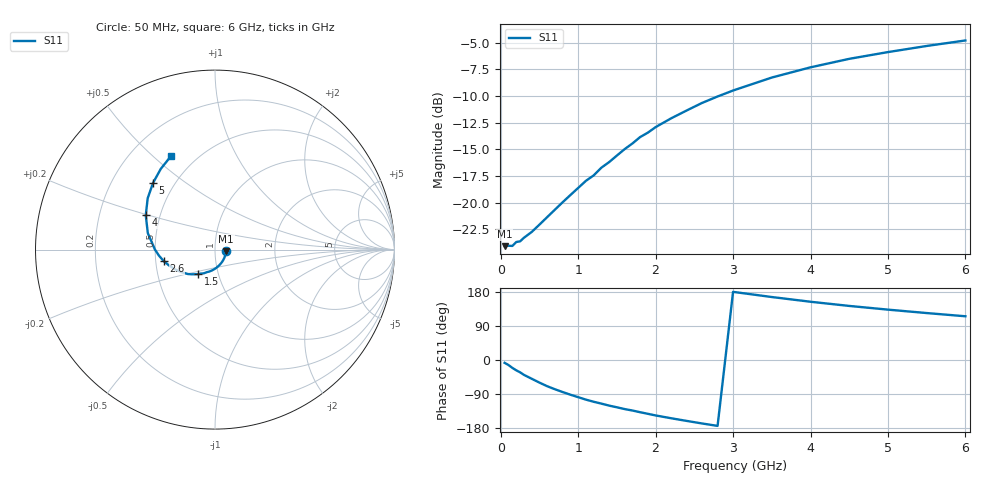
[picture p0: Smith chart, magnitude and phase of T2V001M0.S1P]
! SIEMENS Discrete & RF Semiconductors
! BAS70-04W
! Si Schottky Diode in SOT323
! IF = 1 mA
! S-Parameters:  November  1997
# GHz  S  MA  R  50
!  f  S11
! GHz  MAG  ANG
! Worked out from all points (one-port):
!   34 points, 50 MHz to 6 GHz, reference 50 ohm
!   lowest |S11| = -24.1 dB at 50 MHz (marker M1), VSWR 1.13, Z = 56.6 - j0.928 ohm
!   |S11| at or under -10 dB: start of sweep to 2.82 GHz
!   S11 on the Smith chart (normalised r, x): 50 MHz: 1.13, -0.02; 1.5 GHz: 0.80, -0.22; 2.6 GHz: 0.55, -0.08; 4 GHz: 0.42, +0.19; 5 GHz: 0.38, +0.38; 6 GHz: 0.37, +0.57
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0.05  0.06254 -7.5
0.15  0.06269 -20.8
0.2  0.06541 -27.2
0.25  0.0659 -32.5
0.3  0.06849 -39.3
0.4  0.0729 -49.5
0.6  0.08556 -69.2
0.8  0.1005 -84.6
1.1  0.1266 -104.6
1.2  0.1341 -110.2
1.3  0.1458 -115.1
1.4  0.1549 -120.4
1.5  0.1662 -124.8
1.6  0.1781 -129.5
1.8  0.2028 -137.8
1.9  0.2128 -142.0
2  0.2258 -146.3
2.2  0.2482 -153.7
2.4  0.2701 -160.7
2.6  0.2931 -167.5
2.8  0.3142 -173.9
3  0.3351 179.8
3.5  0.3854 166.2
4  0.4303 153.7
4.5  0.4716 142.7
5  0.5072 132.9
5.5  0.5418 123.9
6  0.575 115.4
